(* Logix 5000 AddOnInstructionDefinition export AMCI_ANG1E_Registration_Move_CCW; software revision 20.03 *)

ADD_ON_INSTRUCTION AMCI_ANG1E_Registration_Move_CCW   (* revision 5.0, vendor AMCI, ExecuteEnableInFalse *)
// Revision note:
// Version 5.0 unlatched the error bit if the rung goes false.
VAR_INPUT
   Type_0_for_standard_1_for_indexed : BOOL;
   Axis_Status_bits : INT; {required}
   slot_axis_number : INT; {required}
   Stopping_Distance : DINT; {required}
   Programmed_Speed : DINT; {required}
   Acceleration : INT; {required}
   Deceleration : INT; {required}
   Minimum_Registration_Move_Distance : DINT; {required}
END_VAR
VAR_IN_OUT
   AMCI_ANG1E_output_data : INT[10]; {required}
END_VAR
VAR_OUTPUT
   EN : BOOL; {access Read Only, visible}
   Registration_Move_CCW_Occurring : BOOL; {access Read Only, visible}
   ER : BOOL; {access Read Only, visible}
END_VAR
VAR
   Upper_Result_X_1000 : DINT;
   command_data_block : INT[10];
        [0]   // Command Bits MSW
        [1]   // Command Bits LSW
        [2]   // Upper Target Position
        [3]   // Lower Target Position
        [4]   // Upper Programmed Speed
        [5]   // Lower Programmed Speed
   index : INT;
END_VAR

ROUTINE EnableInFalse   (* ladder *)
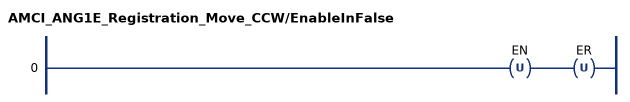
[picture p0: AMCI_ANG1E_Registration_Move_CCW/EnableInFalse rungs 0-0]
   0: OTU(EN)OTU(ER);
END_ROUTINE

ROUTINE Logic   (* ladder *)
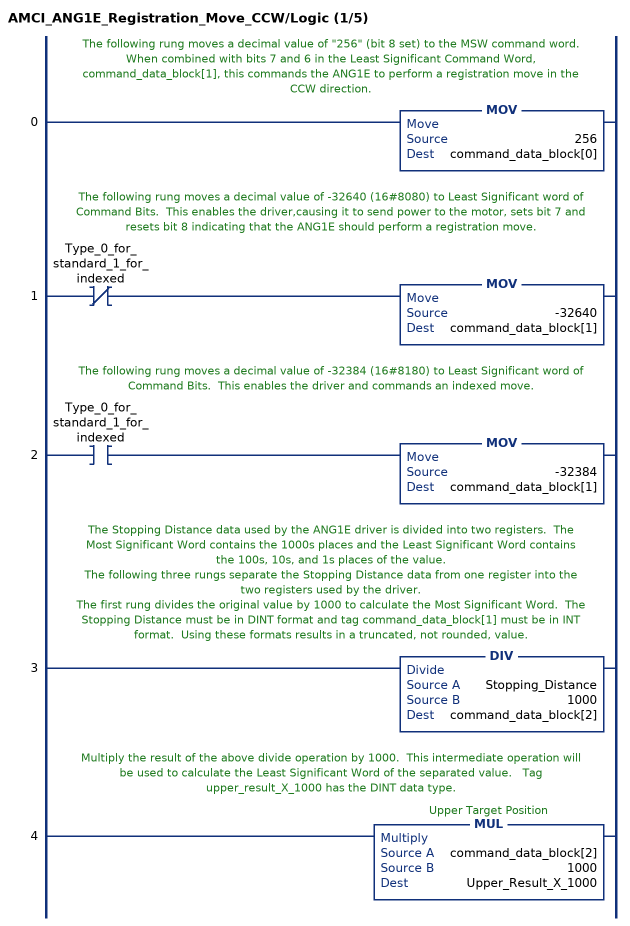
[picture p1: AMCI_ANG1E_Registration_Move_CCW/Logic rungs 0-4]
   // The following rung moves a decimal value of "256" (bit 8 set) to the MSW command word.  When combined with bits 7 and 6 in the Least Significant Command Word, command_data_block[1], this commands the ANG1E to perform a registration move in the CCW direction.
   0: MOV(256,command_data_block[0]);
   // The following rung moves a decimal value of -32640 (16#8080) to Least Significant word of Command Bits.  This enables the driver,causing it to send power to the motor, sets bit 7 and resets bit 8 indicating that the ANG1E should perform a registration move.
   1: XIO(Type_0_for_standard_1_for_indexed)MOV(-32640,command_data_block[1]);
   // The following rung moves a decimal value of -32384 (16#8180) to Least Significant word of Command Bits.  This enables the driver and commands an indexed move.
   2: XIC(Type_0_for_standard_1_for_indexed)MOV(-32384,command_data_block[1]);
   // The Stopping Distance data used by the ANG1E driver is divided into two registers.  The Most Significant Word contains the 1000s places and the Least Significant Word contains the 100s, 10s, and 1s places of the value.
   // The following three rungs separate the Stopping Distance data from one register into the two registers used by the driver.
   // The first rung divides the original value by 1000 to calculate the Most Significant Word.  The Stopping Distance must be in DINT format and tag command_data_block[1] must be in INT format.  Using these formats results in a truncated, not rounded, value.
   3: DIV(Stopping_Distance,1000,command_data_block[2]);
   // Multiply the result of the above divide operation by 1000.  This intermediate operation will be used to calculate the Least Significant Word of the separated value.   Tag upper_result_X_1000 has the DINT data type.
   4: MUL(command_data_block[2],1000,Upper_Result_X_1000);
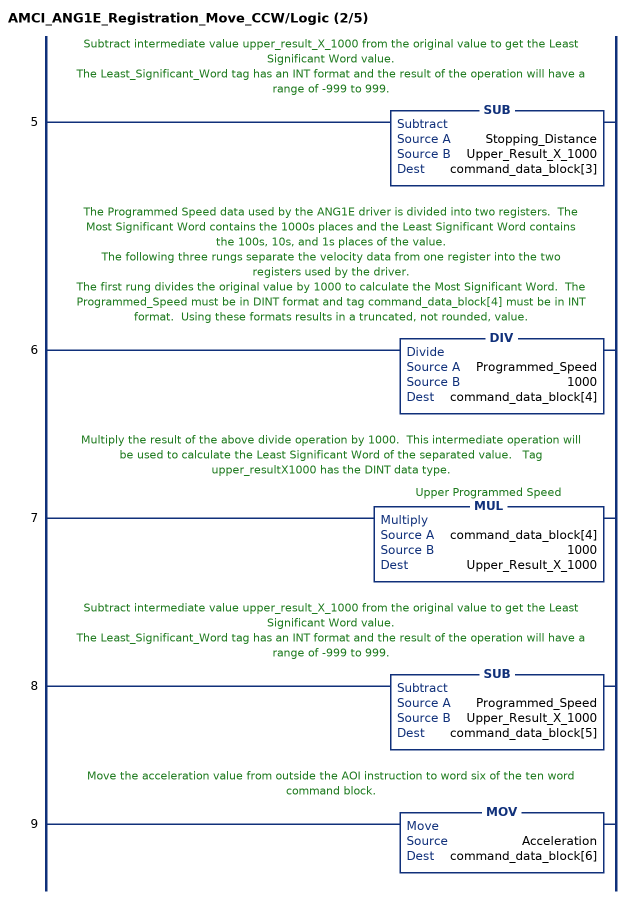
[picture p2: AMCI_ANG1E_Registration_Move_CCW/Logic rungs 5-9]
   // Subtract intermediate value upper_result_X_1000 from the original value to get the Least Significant Word value.
   // The Least_Significant_Word tag has an INT format and the result of the operation will have a range of -999 to 999.
   5: SUB(Stopping_Distance,Upper_Result_X_1000,command_data_block[3]);
   // The Programmed Speed data used by the ANG1E driver is divided into two registers.  The Most Significant Word contains the 1000s places and the Least Significant Word contains the 100s, 10s, and 1s places of the value.
   // The following three rungs separate the velocity data from one register into the two registers used by the driver.
   // The first rung divides the original value by 1000 to calculate the Most Significant Word.  The Programmed_Speed must be in DINT format and tag command_data_block[4] must be in INT format.  Using these formats results in a truncated, not rounded, value.
   6: DIV(Programmed_Speed,1000,command_data_block[4]);
   // Multiply the result of the above divide operation by 1000.  This intermediate operation will be used to calculate the Least Significant Word of the separated value.   Tag upper_resultX1000 has the DINT data type.
   7: MUL(command_data_block[4],1000,Upper_Result_X_1000);
   // Subtract intermediate value upper_result_X_1000 from the original value to get the Least Significant Word value.
   // The Least_Significant_Word tag has an INT format and the result of the operation will have a range of -999 to 999.
   8: SUB(Programmed_Speed,Upper_Result_X_1000,command_data_block[5]);
   // Move the acceleration value from outside the AOI instruction to word six of the ten word command block.
   9: MOV(Acceleration,command_data_block[6]);
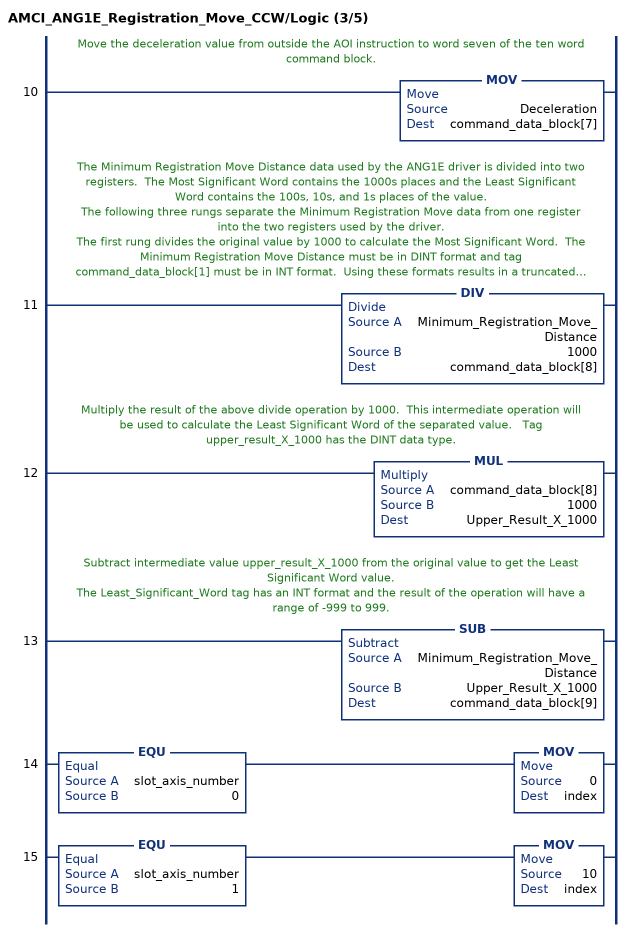
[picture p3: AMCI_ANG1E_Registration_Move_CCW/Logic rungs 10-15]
   // Move the deceleration value from outside the AOI instruction to word seven of the ten word command block.
   10: MOV(Deceleration,command_data_block[7]);
   // The Minimum Registration Move Distance data used by the ANG1E driver is divided into two registers.  The Most Significant Word contains the 1000s places and the Least Significant Word contains the 100s, 10s, and 1s places of the value.
   // The following three rungs separate the Minimum Registration Move data from one register into the two registers used by the driver.
   // The first rung divides the original value by 1000 to calculate the Most Significant Word.  The Minimum Registration Move Distance must be in DINT format and tag command_data_block[1] must be in INT format.  Using these formats results in a truncated, not rounded, value.
   11: DIV(Minimum_Registration_Move_Distance,1000,command_data_block[8]);
   // Multiply the result of the above divide operation by 1000.  This intermediate operation will be used to calculate the Least Significant Word of the separated value.   Tag upper_result_X_1000 has the DINT data type.
   12: MUL(command_data_block[8],1000,Upper_Result_X_1000);
   // Subtract intermediate value upper_result_X_1000 from the original value to get the Least Significant Word value.
   // The Least_Significant_Word tag has an INT format and the result of the operation will have a range of -999 to 999.
   13: SUB(Minimum_Registration_Move_Distance,Upper_Result_X_1000,command_data_block[9]);
   14: EQU(slot_axis_number,0)MOV(0,index);
   15: EQU(slot_axis_number,1)MOV(10,index);
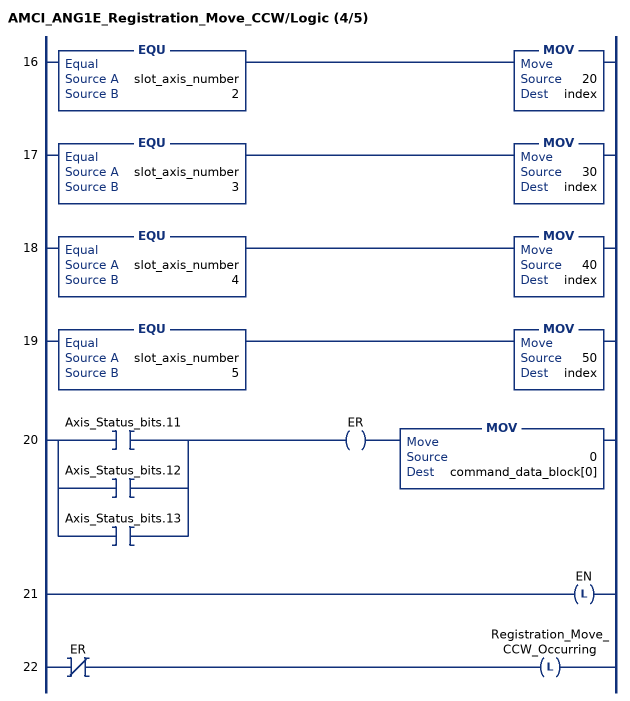
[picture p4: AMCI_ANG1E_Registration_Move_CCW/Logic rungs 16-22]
   16: EQU(slot_axis_number,2)MOV(20,index);
   17: EQU(slot_axis_number,3)MOV(30,index);
   18: EQU(slot_axis_number,4)MOV(40,index);
   19: EQU(slot_axis_number,5)MOV(50,index);
   20: [XIC(Axis_Status_bits.11) ,XIC(Axis_Status_bits.12) ,XIC(Axis_Status_bits.13) ]OTE(ER)MOV(0,command_data_block[0]);
   21: OTL(EN);
   22: XIO(ER)OTL(Registration_Move_CCW_Occurring);
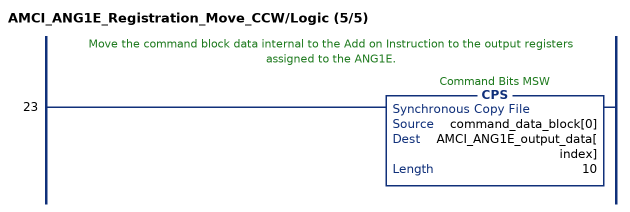
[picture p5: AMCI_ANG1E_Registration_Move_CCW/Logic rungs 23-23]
   // Move the command block data internal to the Add on Instruction to the output registers assigned to the ANG1E.
   23: CPS(command_data_block[0],AMCI_ANG1E_output_data[index],10);
END_ROUTINE
END_ADD_ON_INSTRUCTION
